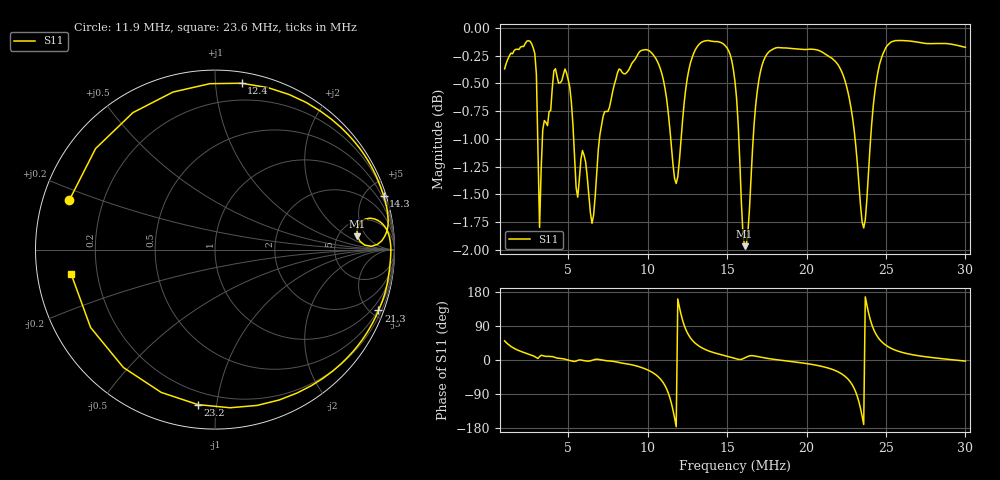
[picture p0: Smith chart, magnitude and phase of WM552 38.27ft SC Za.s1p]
!Created via Zplots "Save as S1P" button
!Original data file:  $remote$.s1p
!Transmission line transform:  None
# MHZ S MA R 50
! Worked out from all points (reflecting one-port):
!   291 points, 1 MHz to 30 MHz, reference 50 ohm
!   lowest |S11| = -2.0 dB at 16.1 MHz (marker M1), VSWR 8.87, Z = 379 + j156 ohm
!   phase of S11 starts at 51 deg and turns -773 deg over the sweep
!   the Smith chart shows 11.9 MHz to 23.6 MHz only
!   S11 on the Smith chart (normalised r, x): 11.9 MHz: 0.08, +0.17; 12.4 MHz: 0.08, +1.17; 14.3 MHz: 0.30, +6.40; 21.3 MHz: 0.45, -5.51; 23.2 MHz: 0.13, -0.89; 23.6 MHz: 0.10, -0.08
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1  0.9584 50.6
2  0.9803 23.1
3.1  0.8823 3.9
4.7  0.9528 3.2
8.3  0.9575 -7.6
10.4  0.9714 -35.4
10.9  0.9534 -55.0
11.3  0.9156 -87.0
11.6  0.8675 -132.7
11.9  0.8569 161.1
12.1  0.8897 120.9
12.4  0.9387 80.9
13.1  0.9802 40.8
14.3  0.9859 17.7
15.5  0.9456 4.2
16.1  0.7974 5.4
19.2  0.9786 -4.9
21.3  0.972 -20.4
22.8  0.9204 -60.3
23.2  0.8688 -96.3
23.4  0.8318 -127.9
23.6  0.8126 -170.2
23.9  0.8605 125.2
24.1  0.9048 94.8
24.4  0.9466 66.3
24.9  0.9766 41.9
26.4  0.9866 16.2
30  0.9801 -2.9
